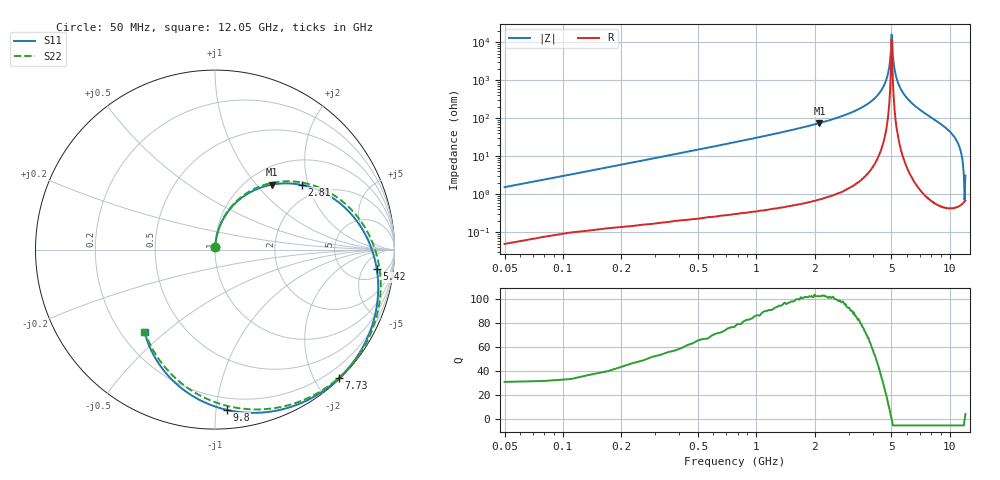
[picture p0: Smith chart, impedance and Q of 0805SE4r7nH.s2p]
! AVX Thin Film Operation		Date: May 2002
! Description: Accu-L® Series, Thin Film, SMD, RF Inductors
! Part Number: L08054R7CEWTR
! 50 MHz  -  12.05 GHz
! Serial Measurements
# mhz S db R 50
!	S11		S21		S12		S22
!	dB	Phase	dB	Phase	dB	Phase	dB	Phase
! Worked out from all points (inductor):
!   401 points, 50 MHz to 12.05 GHz, reference 50 ohm
!   read as 1/Y11, port 2 shorted: L = 4.74 nH near 110 MHz
!   highest Q = 102 at 2.12 GHz (marker M1), where L = 5.56 nH
!   self-resonance near 5 GHz
!   S11 on the Smith chart (normalised r, x): 50 MHz: 1.00, +0.03; 2.81 GHz: 1.61, +1.82; 5.42 GHz: 8, -10; 7.73 GHz: 0.02, -2.35; 9.8 GHz: 0.12, -1.07; 12.05 GHz: 0.29, -0.43
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50  -37.70 86.7  -0.00 -1.0  -0.00 -1.0  -37.70 86.7
260  -23.75 83.5  -0.03 -5.1  -0.03 -5.1  -23.75 83.6
590  -16.77 77.4  -0.11 -11.4  -0.11 -11.4  -16.77 77.8
1190  -10.90 66.1  -0.40 -22.8  -0.40 -22.8  -10.90 66.9
2060  -6.58 50.0  -1.12 -38.8  -1.12 -38.8  -6.58 51.3
2120  -6.37 48.9  -1.19 -39.9  -1.19 -39.9  -6.37 50.3
2810  -4.38 36.6  -2.03 -52.0  -2.03 -52.0  -4.38 38.5
4070  -2.15 15.2  -4.18 -73.0  -4.18 -73.0  -2.15 17.9
5420  -0.84 -6.9  -7.78 -94.6  -7.78 -94.6  -0.84 -3.4
6050  -0.46 -17.3  -10.38 -104.5  -10.38 -104.5  -0.46 -13.3
6740  -0.18 -28.8  -14.86 -115.4  -14.86 -115.4  -0.18 -24.5
7220  -0.08 -37.1  -20.77 -122.3  -20.77 -122.3  -0.08 -32.5
7460  -0.05 -41.3  -26.82 -123.8  -26.82 -123.8  -0.05 -36.7
7670  -0.04 -45.0  -41.38 -52.3  -41.38 -52.3  -0.04 -40.3
7730  -0.04 -46.1  -40.53 -6.2  -40.53 -6.2  -0.04 -41.4
7880  -0.05 -48.8  -28.55 37.0  -28.55 37.0  -0.05 -44.0
8060  -0.07 -52.1  -22.68 37.1  -22.68 37.1  -0.07 -47.3
8690  -0.23 -63.9  -13.87 27.3  -13.87 27.3  -0.23 -59.0
9800  -0.96 -85.8  -7.30 5.8  -7.30 5.8  -0.97 -81.2
10070  -1.23 -91.3  -6.30 0.3  -6.30 0.3  -1.24 -86.8
11090  -2.63 -111.9  -3.57 -21.0  -3.57 -21.0  -2.65 -109.0
12050  -4.37 -130.4  -2.09 -41.0  -2.09 -41.0  -4.40 -130.7
